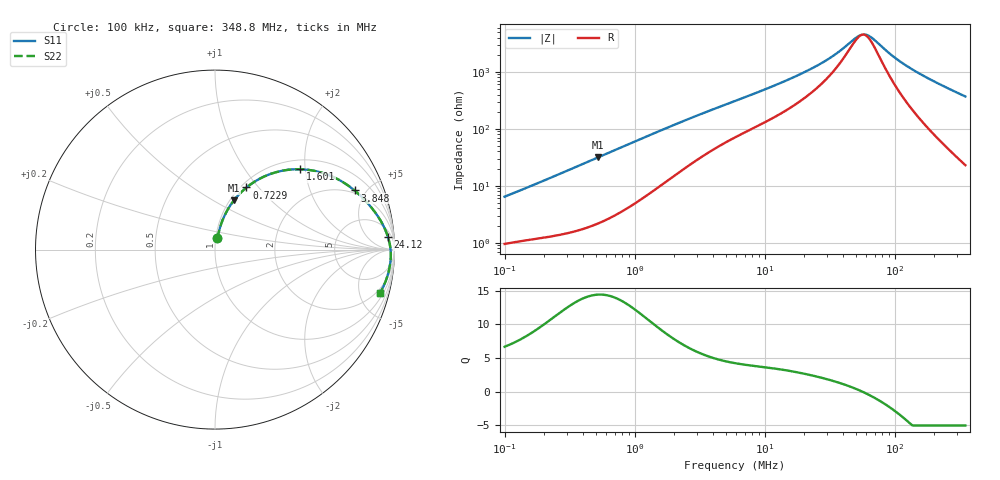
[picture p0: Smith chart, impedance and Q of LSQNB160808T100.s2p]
! LSQNB160808T100  S-PARAMETER MODEL  ( General Type )
! Model Generated by TAIYO YUDEN Corporation (http://www.ty-top.com)
! Version 2.0
! TAIYO YUDEN Control No. 100810NF25SB-FKC
! Copyright(c) 2007 TAIYO YUDEN CO.,LTD. All Rights Reserved.
! Product Description (link to TY-COMPAS)
! https://ds.yuden.co.jp/TYCOMPAS/or/detail?pn=LSQNB160808T100K&u=M
! Products Name : Inductors
! Characteristics :
!  Inductance : 10 uH , SRF(min) : 32 MHz , DC Resistance(max) : 0.468 Ohm
!  Rated Current : Saturation :115 mA , Temp Rise : 380 mA (40 degC)
!  Case Size : 1.6 x 0.8 / 0.063 x 0.031 [mm/inch] , Thickness : 0.8 / 0.031 [mm/inch]
!  (Conditions: Temperature = 25 degC , DC Bias Current/Voltage = 0A / 0V)
! External Node Assignments :
!  1  o---GGG---o  2
! GND o---------o GND
! Frequency Range : 0.1MHz  -  348.750116MHz  [ 402 STEP ]
# MHz S RI R 50
! Freq[MHz].  S11 Real  S11 Imag  S21 Real  S21 Imag  S12 Real  S12 Imag  S22 Real  S22 Imag
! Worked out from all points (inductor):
!   401 points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, 100 kHz to 348.8 MHz, reference 50 ohm
!   read as one part in series: L = 9.95 uH near 104.2 kHz
!   highest Q = 14.4 at 521.6 kHz (marker M1), where L = 9.57 uH
!   self-resonance near 56.51 MHz
!   S11 on the Smith chart (normalised r, x): 100 kHz: 1.02, +0.13; 722.9 kHz: 1.06, +0.87; 1.601 MHz: 1.20, +1.88; 3.848 MHz: 1.81, +4.17; 24.12 MHz: 11, +22; 348.8 MHz: 1.46, -7.37
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0.1  0.0134 0.0623  0.9866 -0.0623  0.9866 -0.0623  0.0134 0.0623
0.208366  0.0277 0.1224  0.9723 -0.1224  0.9723 -0.1224  0.0277 0.1224
0.392077  0.0673 0.2169  0.9327 -0.2169  0.9327 -0.2169  0.0673 0.2169
0.521626  0.1055 0.2745  0.8945 -0.2745  0.8945 -0.2745  0.1055 0.2745
0.722869  0.1755 0.346  0.8245 -0.346  0.8245 -0.346  0.1755 0.346
1.08689  0.3106 0.422  0.6894 -0.422  0.6894 -0.422  0.3106 0.422
1.537242  0.4566 0.4479  0.5434 -0.4479  0.5434 -0.4479  0.4566 0.4479
1.601234  0.4743 0.4477  0.5257 -0.4477  0.5257 -0.4477  0.4743 0.4477
2.559467  0.6613 0.4035  0.3387 -0.4035  0.3387 -0.4035  0.6613 0.4035
3.848355  0.7775 0.3297  0.2225 -0.3297  0.2225 -0.3297  0.7775 0.3297
5.905507  0.8566 0.2519  0.1434 -0.2519  0.1434 -0.2519  0.8566 0.2519
12.55856  0.934 0.141  0.066 -0.141  0.066 -0.141  0.934 0.141
23.15412  0.9622 0.0745  0.0378 -0.0745  0.0378 -0.0745  0.9622 0.0745
24.11798  0.9634 0.0707  0.0366 -0.0707  0.0366 -0.0707  0.9634 0.0707
34.11126  0.9715 0.0407  0.0285 -0.0407  0.0285 -0.0407  0.9715 0.0407
51.28891  0.9774 0.00787  0.0226 -0.00787  0.0226 -0.00787  0.9774 0.00787
56.79432  0.9783 -0.000409  0.0217 0.000409  0.0217 0.000409  0.9783 -0.000409
65.50869  0.9792 -0.0123  0.0208 0.0123  0.0208 0.0123  0.9792 -0.0123
90.78195  0.9795 -0.0416  0.0205 0.0416  0.0205 0.0416  0.9795 -0.0416
115.9511  0.9776 -0.0666  0.0224 0.0666  0.0224 0.0666  0.9776 -0.0666
157.4415  0.9718 -0.1036  0.0282 0.1036  0.0282 0.1036  0.9718 -0.1036
348.7501  0.9185 -0.2442  0.0815 0.2442  0.0815 0.2442  0.9185 -0.2442
